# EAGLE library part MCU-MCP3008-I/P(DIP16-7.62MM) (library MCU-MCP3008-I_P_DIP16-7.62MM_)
310990040
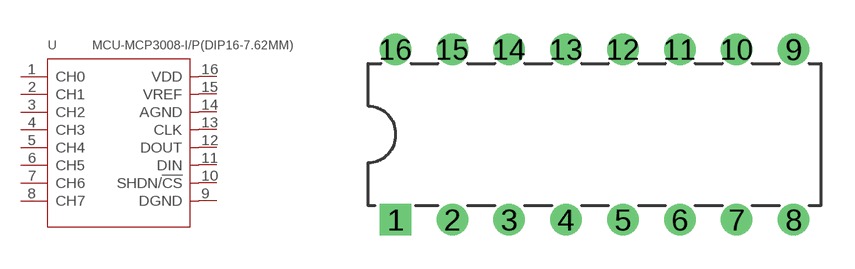
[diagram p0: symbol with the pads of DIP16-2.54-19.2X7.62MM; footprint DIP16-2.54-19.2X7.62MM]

Designator prefix U

## MCU-MCP3008-I/P(DIP16-7.62MM) (Availability: Good; Description: 8 Channel SPI Serial Interface 2.7 V 10-Bit A/D Converter Through Hole - PDIP-16; MF: Microchip; MP: MCP3008-I/P; Package: DIP-16 Microchip; Price: 2.16 USD)  [DIP16-2.54-19.2X7.62MM]
1  CH0  out
2  CH1  in
3  CH2  out
4  CH3  in
5  CH4  in
6  CH5  in
7  CH6  out
8  CH7  in
9  DGND  out
10  SHDN/!CS  out
11  DIN  in
12  DOUT  in
13  CLK  out
14  AGND  in
15  VREF  in
16  VDD  sup

## Footprint DIP16-2.54-19.2X7.62MM (pad centres in mm)
drill 0.9 pad 1.4 square: 1 -8.89,-3.81
drill 0.9 pad 1.4: 2 -6.35,-3.81; 3 -3.81,-3.81; 4 -1.27,-3.81; 5 1.27,-3.81; 6 3.81,-3.81; 7 6.35,-3.81; 8 8.89,-3.81; 9 8.89,3.81; 10 6.35,3.81; 11 3.81,3.81; 12 1.27,3.81; 13 -1.27,3.81; 14 -3.81,3.81; 15 -6.35,3.81; 16 -8.89,3.81

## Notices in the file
This work is licensed under a Creative Commons Attribution-ShareAlike 4.0 International License (CC BY-SA) with Design Exception 1.0
